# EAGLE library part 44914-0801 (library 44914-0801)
Micro-Fit CPI Header, Compliant Pin Interface, Dual Row, Vertical, 8 Circuits, Tin (Sn) Plating, Glow-Wire Capable Source: Datasheet
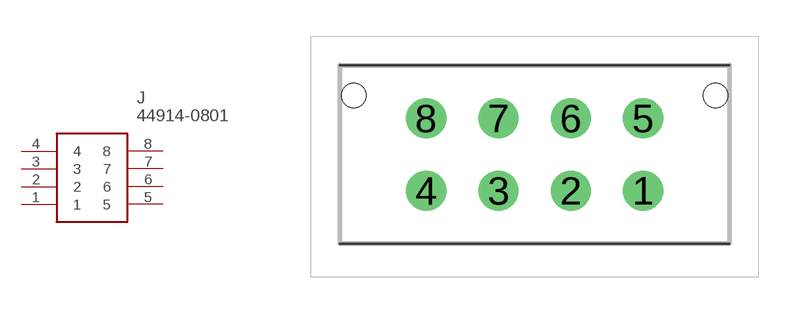
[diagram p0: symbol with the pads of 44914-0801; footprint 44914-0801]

Designator prefix J

## 44914-0801 (Description: Micro-Fit CPI Header, Compliant Pin Interface, Dual Row, Vertical, 8 Circuits, Tin (Sn) Plating, Glow-Wire Capable; Height: mm; Manufacturer_Name: Molex; Manufacturer_Part_Number: 44914-0801; Mouser_Part_Number: 538-44914-0801; Mouser_Price-Stock: https://www.mouser.co.uk/ProductDetail/Molex/44914-0801?qs=c7kbnNtxOmhgMCdedRAzWQ%3D%3D)  [44914-0801]
1  1
2  2
3  3
4  4
5  5
6  6
7  7
8  8

## Footprint 44914-0801 (pad centres in mm)
44914-0801
drill 1.11 pad 1.65: 1 0,0; 2 -3,0; 3 -6,0; 4 -9,0; 5 0,3; 6 -3,3; 7 -6,3; 8 -9,3
hole 1.02 at 3,3.94
hole 1.02 at -12,3.94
